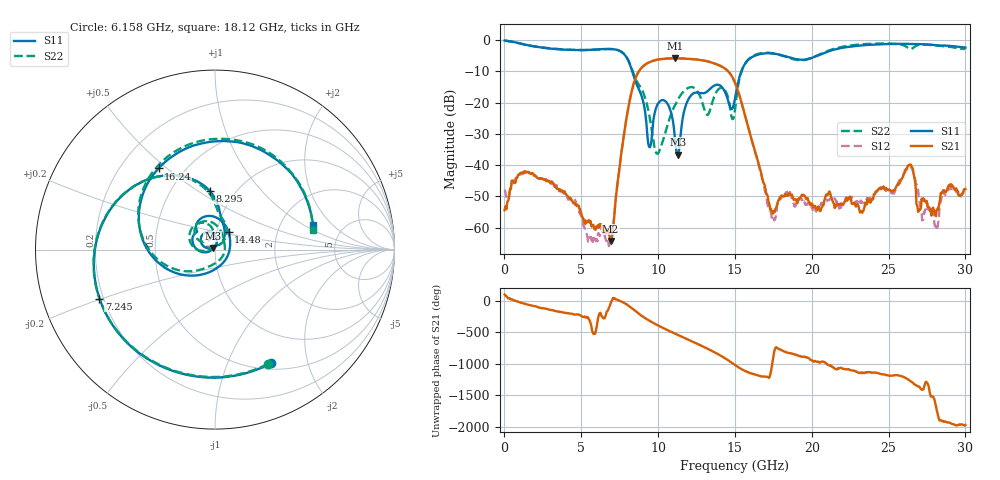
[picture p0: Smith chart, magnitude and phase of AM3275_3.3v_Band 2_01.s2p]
!Keysight Technologies,N5245B,MY58422270,A.16.20.02
!Date: Thursday, March 27, 2025 01:52:06
!Correction: S11(C  2-Port  )
!S21(C  2-Port  )
!S12(C  2-Port  )
!S22(C  2-Port  )
!S2P File: Measurements: S11, S21, S12, S22:
# Hz S  dB  R 50
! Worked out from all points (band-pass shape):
!   801 points, 10 MHz to 30 GHz, reference 50 ohm
!   highest |S21| = -5.89 dB at 11.11 GHz (marker M1); lowest = -64.2 dB at 6.908 GHz (marker M2)
!   |S21| within 3 dB of the highest: 8.929 GHz to 14.27 GHz (5.343 GHz wide, 46.1 % of centre)
!   lowest |S11| = -36.6 dB at 11.29 GHz (marker M3), VSWR 1.03, Z = 48.8 + j0.835 ohm
!   |S11| at or under -10 dB: 8.315 GHz to 15.42 GHz (7.107 GHz wide, 59.9 % of centre)
!   |S22| runs from -36.4 to -0.2 dB; largest |S21 - S12| = 0.0057
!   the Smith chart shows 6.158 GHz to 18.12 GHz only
!   S11 on the Smith chart (normalised r, x): 6.158 GHz: 0.57, -1.45; 7.245 GHz: 0.18, -0.20; 8.295 GHz: 0.77, +0.56; 14.48 GHz: 1.14, +0.22; 16.24 GHz: 0.36, +0.47; 18.12 GHz: 3.03, +1.24
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1e7  -0.23 -5.7  -54.34 102.7  -47.79 -35.3  -0.20 -6.1
8.722125e8  -0.98 -87.1  -43.35 -9.3  -43.17 -8.3  -0.99 -87.0
1.996838e9  -2.14 -171.4  -43.29 -84.2  -43.52 -85.6  -2.14 -171.4
3.533825e9  -3.02 100.9  -47.77 -171.2  -47.14 -162.7  -2.95 100.5
5.033325e9  -3.29 14.8  -56.28 117.7  -56.60 122.9  -3.25 13.5
6.15795e9  -3.02 -63.8  -59.20 142.5  -62.20 -129.0  -3.07 -65.2
6.9077e9  -2.91 -126.0  -64.21 -38.6  -63.88 163.1  -2.94 -126.6
7.245088e9  -3.11 -157.1  -50.48 24.2  -50.98 30.8  -3.11 -157.2
8.294738e9  -9.68 95.1  -16.13 -115.2  -16.16 -115.5  -9.36 98.8
9.419362e9  -34.16 101.6  -7.18 48.0  -7.16 47.9  -23.85 44.8
1.001916e10  -20.17 144.6  -6.26 -32.0  -6.27 -32.2  -36.15 125.7
1.11063e10  -32.01 81.0  -5.89 -160.1  -5.89 -160.2  -20.75 -178.2
1.129374e10  -36.60 144.6  -5.90 178.9  -5.90 178.7  -18.98 175.9
1.283072e10  -17.06 135.9  -6.49 6.2  -6.49 6.1  -19.33 96.1
1.448018e10  -18.20 52.2  -9.65 149.0  -9.64 148.9  -17.33 86.9
1.5005e10  -18.74 -94.6  -13.68 61.0  -13.67 60.9  -22.43 -88.2
1.624209e10  -5.18 124.8  -34.48 -86.4  -34.61 -88.1  -4.96 124.4
1.811646e10  -4.98 14.3  -49.82 -74.0  -50.35 -65.0  -5.09 11.4
2.002832e10  -5.73 -136.7  -52.25 132.4  -53.88 149.8  -5.65 -141.1
2.246501e10  -2.20 104.2  -50.83 -13.6  -50.10 -14.0  -1.84 104.1
2.501416e10  -1.34 38.3  -48.06 -105.0  -48.39 -107.8  -1.17 35.8
3e10  -2.47 -110.3  -47.64 -175.2  -48.28 -155.3  -2.86 -109.6
